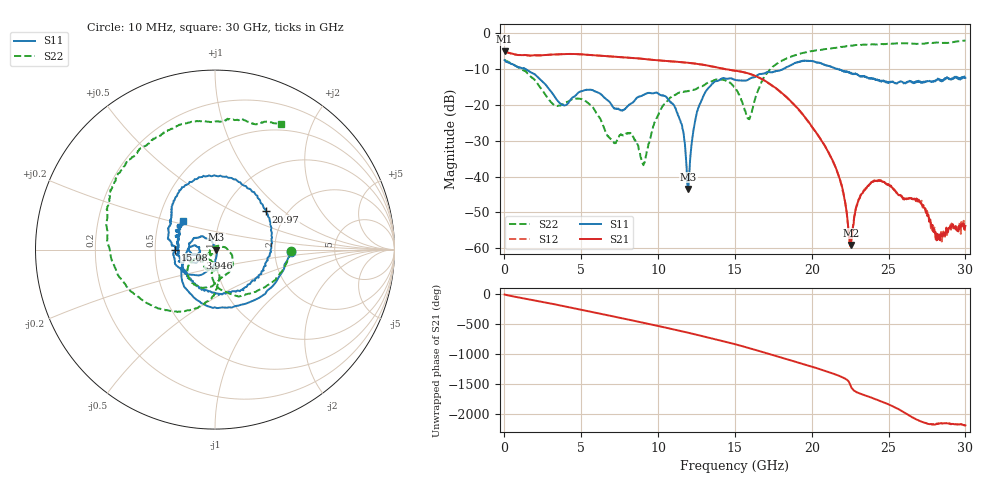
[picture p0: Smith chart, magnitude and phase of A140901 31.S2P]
!  2-Port S-parameters saved by WinCal
! VAR MeasName=S-Parameters (CALIBRATED_DATA) read from VNA (N5244A)
! VAR MeasDate=11/3/2014 9:29:20 AM
! VAR NAME=A140901 31
! VAR FILENAME=A140901 31.S2P
! VAR DATE=11/3/2014 9:29:20 AM
! VAR PHYS_PORTS=1,2
# Hz S RI R 50
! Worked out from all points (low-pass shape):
!   801 points, 10 MHz to 30 GHz, reference 50 ohm
!   highest |S21| = -5.06 dB at 10 MHz (marker M1); lowest = -59.1 dB at 22.54 GHz (marker M2)
!   |S21| within 3 dB of the highest: start of sweep to 11.45 GHz
!   lowest |S11| = -43.5 dB at 11.97 GHz (marker M3), VSWR 1.01, Z = 50.7 + j0.0151 ohm
!   |S11| at or under -10 dB: 1.375 GHz to 18.15 GHz (16.77 GHz wide, 172 % of centre); 21.67 GHz to end of sweep
!   |S22| runs from -36.8 to -2.0 dB; largest |S21 - S12| = 0.0035
!   S11 on the Smith chart (normalised r, x): 10 MHz: 2.45, -0.07; 3.946 GHz: 0.84, -0.08; 15.08 GHz: 0.64, -0.00; 20.97 GHz: 1.56, +0.76; 30 GHz: 0.67, +0.23
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1e7  0.4207 -0.0112  0.5583 -0.0086  0.5571 -0.00853  0.4235 -0.00681
1.921862e9  -0.1637 -0.216  -0.0601 -0.4886  -0.0602 -0.4885  0.0355 -0.2243
3.946188e9  -0.0863 -0.0476  -0.4817 0.1752  -0.4814 0.1749  0.00827 -0.1073
5.033325e9  -0.1411 -0.0655  -0.1018 0.496  -0.1014 0.4958  -0.0475 -0.1104
6.945188e9  -0.1007 0.0168  0.4745 -0.00153  0.4742 -0.00147  -0.0229 -0.0244
8.219762e9  -0.0992 -0.0316  0.1629 -0.4242  0.1622 -0.4238  -0.0269 -0.0295
9.007e9  -0.136 -0.0164  -0.1677 -0.405  -0.1673 -0.4051  -0.00991 0.0113
1.001916e10  -0.1389 0.0389  -0.4103 -0.0824  -0.4103 -0.0816  0.0723 -0.00339
1.14062e10  -0.0278 0.056  -0.1473 0.3673  -0.1463 0.3668  0.0776 -0.1275
1.196851e10  0.00667 0.000149  0.0776 0.3787  0.0781 0.3775  0.0447 -0.1489
1.298068e10  -0.0537 -0.1269  0.3471 0.0996  0.3473 0.0997  0.00246 -0.1867
1.5005e10  -0.2236 -0.00484  -0.1173 -0.2762  -0.1186 -0.2742  -0.1469 -0.0897
1.507998e10  -0.2209 -0.00102  -0.1407 -0.2635  -0.1417 -0.2614  -0.1443 -0.0816
1.59047e10  -0.2264 0.0203  -0.2732 -0.0144  -0.2732 -0.0128  -0.0292 -0.058
1.729174e10  -0.257 0.1272  0.0399 0.1911  0.0409 0.1894  -0.0668 -0.3044
2.002832e10  0.0928 0.3991  -0.0328 -0.0364  -0.0322 -0.0367  -0.5514 -0.1137
2.096551e10  0.2826 0.2123  -0.0213 0.0115  -0.0215 0.0109  -0.5998 0.0565
2.253999e10  0.2232 -0.1727  -3.59e-05 -0.00111  -0.000109 -0.00114  -0.5728 0.3449
2.336471e10  0.0385 -0.2491  -0.00286 0.00551  -0.00293 0.00546  -0.4907 0.4908
2.501416e10  -0.1638 -0.1182  0.00564 -0.00527  0.00564 -0.00531  -0.2744 0.6588
2.82006e10  -0.2201 0.0769  0.00131 -8.64e-05  0.00146 -8e-05  0.1571 0.7246
3e10  -0.1767 0.1602  0.00169 -0.00115  0.00172 -0.000984  0.367 0.7012
